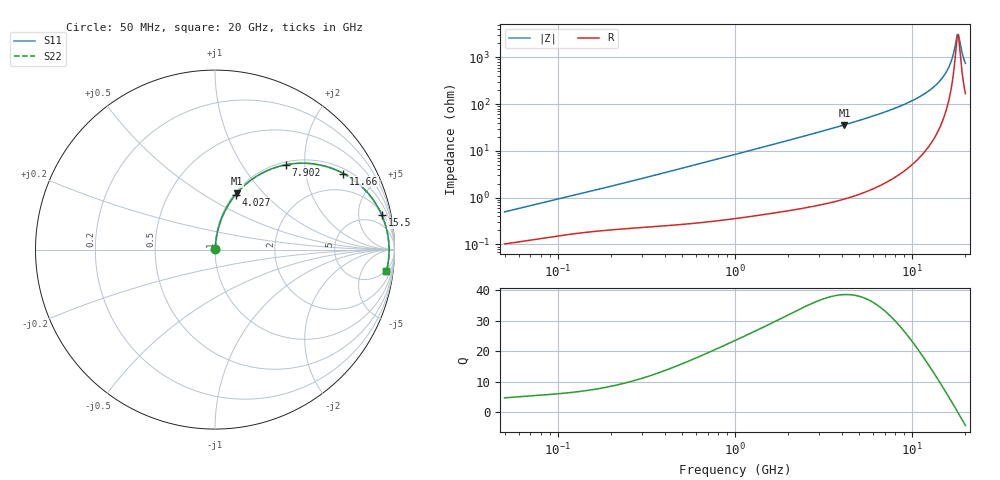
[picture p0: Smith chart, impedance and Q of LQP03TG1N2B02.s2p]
!Murata Part Number: LQP03TG1N2B02
!These Parameters are Measured in Series Mode Connection
!  o--[Z]--o
!Port1  Port2
!  o-------o
!Freq. Start=50[MHz] Stop=20[GHz], 401[Steps]
# Hz S RI R 50
!Freq.(Hz) S11(Real) S11(Imag) S21(Real) S21(Imag) S12(Real) S12(Imag) S22(Real) S22(Imag)
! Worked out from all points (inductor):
!   401 points, 50 MHz to 20 GHz, reference 50 ohm
!   read as one part in series: L = 1.52 nH near 51.52 MHz
!   highest Q = 38.6 at 4.149 GHz (marker M1), where L = 1.38 nH
!   self-resonance near 18.01 GHz
!   S11 on the Smith chart (normalised r, x): 50 MHz: 1.00, +0.01; 4.027 GHz: 1.02, +0.70; 7.902 GHz: 1.05, +1.60; 11.66 GHz: 1.18, +3.25; 15.5 GHz: 2.39, +9.23; 20 GHz: 4, -14
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5e7  0.00105 0.00485  0.999 -0.00485  0.999 -0.00485  0.00105 0.00485
1.364002e8  0.00192 0.0122  0.9981 -0.0122  0.9981 -0.0122  0.00192 0.0122
3.721004e8  0.00343 0.0315  0.9966 -0.0315  0.9966 -0.0315  0.00343 0.0315
1e9  0.0105 0.0826  0.9895 -0.0826  0.9895 -0.0826  0.0105 0.0826
2.728004e9  0.0558 0.2159  0.9442 -0.2159  0.9442 -0.2159  0.0558 0.2159
4.026975e9  0.1144 0.3056  0.8856 -0.3056  0.8856 -0.3056  0.1144 0.3056
4.149438e9  0.121 0.3134  0.879 -0.3134  0.879 -0.3134  0.121 0.3134
5.683258e9  0.2175 0.3992  0.7825 -0.3992  0.7825 -0.3992  0.2175 0.3992
7.442007e9  0.3546 0.4629  0.6454 -0.4629  0.6454 -0.4629  0.3546 0.4629
7.901521e9  0.3936 0.4724  0.6064 -0.4724  0.6064 -0.4724  0.3936 0.4724
9.745021e9  0.5555 0.4766  0.4445 -0.4766  0.4445 -0.4766  0.5555 0.4766
1.166392e10  0.7155 0.424  0.2845 -0.424  0.2845 -0.424  0.7155 0.424
1.375312e10  0.8545 0.3118  0.1455 -0.3118  0.1455 -0.3118  0.8545 0.3118
1.550395e10  0.9299 0.1909  0.0701 -0.1909  0.0701 -0.1909  0.9299 0.1909
1.621653e10  0.9491 0.1388  0.0509 -0.1388  0.0509 -0.1388  0.9491 0.1388
1.670968e10  0.9585 0.1026  0.0415 -0.1026  0.0415 -0.1026  0.9585 0.1026
1.774144e10  0.969 0.0279  0.031 -0.0279  0.031 -0.0279  0.969 0.0279
1.800918e10  0.9698 0.00901  0.0302 -0.00901  0.0302 -0.00901  0.9698 0.00901
1.828096e10  0.9699 -0.00993  0.0301 0.00993  0.0301 0.00993  0.9699 -0.00993
1.855685e10  0.9692 -0.0289  0.0308 0.0289  0.0308 0.0289  0.9692 -0.0289
1.940974e10  0.9627 -0.0852  0.0373 0.0852  0.0373 0.0852  0.9627 -0.0852
2e10  0.9548 -0.1219  0.0452 0.1219  0.0452 0.1219  0.9548 -0.1219
